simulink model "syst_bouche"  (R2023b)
settings: Solver=FixedStepAuto  StartTime=0.0  StopTime=15  FixedStep=0.0001  RelTol=1e-3
libraries: fl_lib x15, nesl_utility x9, ee_lib x1, sdl_lib x1

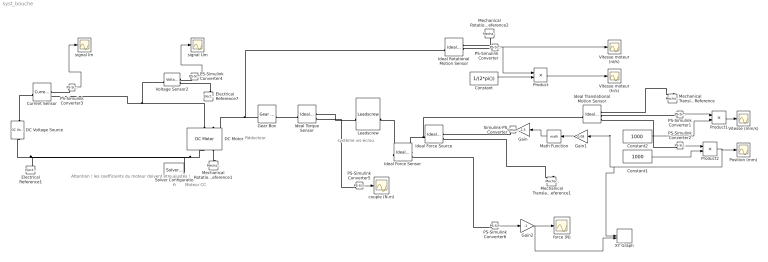
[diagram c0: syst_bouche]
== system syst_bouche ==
  note: Attention ! les coefficients du moteur doivent être ajustés !
  note: système vis-écrou
  note: Moteur CC
  note: Réducteur
  Constant : Constant  Value=1/(2*pi())
  Constant1 : Constant  Value=1000
  Constant2 : Constant  Value=1000
  Current Sensor : fl_lib/Electrical/Electrical Sensors/Current Sensor
  DC Motor : ee_lib/Electromechanical/Brushed Motors/DC Motor  field_option=ee.enum.field_option.pm  Rf=100 Ohm  Lf=1 H  Laf=0.15 H  If0=0 A  parameterization=ee.enum.dcparam_option.circuit_param  Ra=2.22 Ohm  La=0.1e-3 H  emf_or_torque=ee.enum.emf_or_torque.kv  Kv=0.0113 V/(rad/s)  Ki=0.01 N*m/A  T_stall=0.24e-3 N*m  w_max=19100 rpm  w_rated=15000 rpm  P_rated=0.08 W  V_rated=1.5 V  lam_param=ee.enum.lam_param.damping  i_noload=0 A  V_i_noload=1.5 V  J=50 g*cm^2  lam=0.0000015 N*m/(rad/s)  speed0=0 rpm  enable_fault_armature=simscape.enum.onoff.off  rev_faulted=1 / 3  G_faulted_armature=1e-5 S  fault_trigger_armature=ee.enum.faults.faultTrigger.temporal  t_fault_armature=1 s  max_permissible_current_armature=inf A  t_fail_on_current_armature=1 s  enable_fault_field=simscape.enum.onoff.off  G_faulted_field=1e-5 S  fault_trigger_field=ee.enum.faults.faultTrigger.temporal  t_fault_field=1 s  max_permissible_current_field=inf A  t_fail_on_current_field=1 s  fault_action=simscape.enum.assert.action.none  alpha=3.93e-3 1/K  Tmeas=25 degC  thermal_mass=100 J/K  initial_temperature=25 degC
  DC Voltage Source : fl_lib/Electrical/Electrical Sources/DC Voltage Source  v0=12 V
  Electrical Reference1 : fl_lib/Electrical/Electrical Elements/Electrical Reference
  Electrical Reference7 : fl_lib/Electrical/Electrical Elements/Electrical Reference
  Gain : Gain  Gain=2.3
  Gain1 : Gain  Gain=0.08
  Gain2 : Gain  Gain=-1
  Gear Box : fl_lib/Mechanical/Mechanisms/Gear Box  ratio=1  t_in_specify=off  t_in_priority=None  t_in=0 N*m  t_in_nominal_specify=off  t_in_nominal_unit=N*m  t_in_nominal_value=1  t_out_specify=off  t_out_priority=None  t_out=0 N*m  t_out_nominal_specify=off  t_out_nominal_unit=N*m  t_out_nominal_value=1
  Ideal Force Sensor : fl_lib/Mechanical/Mechanical Sensors/Ideal Force Sensor
  Ideal Force Source : fl_lib/Mechanical/Mechanical Sources/Ideal Force Source
  Ideal Rotational Motion Sensor : fl_lib/Mechanical/Mechanical Sensors/Ideal Rotational Motion Sensor  reference=foundation.enum.MeasurementReference.difference  acceleration_port=false  velocity_port=true  position_port=true  wrap_angle=simscape.enum.onoff.off  offset=0 rad
  Ideal Torque Sensor : fl_lib/Mechanical/Mechanical Sensors/Ideal Torque Sensor
  Ideal Translational Motion Sensor : fl_lib/Mechanical/Mechanical Sensors/Ideal Translational Motion Sensor  reference=foundation.enum.MeasurementReference.difference  acceleration_port=false  velocity_port=true  position_port=true  offset=0 m
  Leadscrew : sdl_lib/Gears/Rotational- Translational/Leadscrew  Lead=0 mm  helix_type=sdl.enum.handedness.right  friction_model=sdl.enum.gear_friction.constant  friction_parameterization=sdl.enum.frictionParameterization.geometry  lambda=15 deg  alpha=14.5 deg  fr_coeff=0.08  eff_sn=0.75  eff_ns=0.45  temperature_TLU=[280, 300, 320] K  efficiency_sn_TLU=[.75, .65, .6]  efficiency_ns_TLU=[.5, .45, .4]  pwr_thr=0.001 W  mu_visc=0 N*m/(rad/s)  thermal_mass=50 J/K  temperature_specify=off  temperature_priority=High  temperature=300 K  temperature_nominal_specify=off  temperature_nominal_unit=K  temperature_nominal_value=1
  Math Function : Math
  Mechanical Rotational Reference1 : fl_lib/Mechanical/Rotational Elements/Mechanical Rotational Reference
  Mechanical Rotational Reference2 : fl_lib/Mechanical/Rotational Elements/Mechanical Rotational Reference
  Mechanical Translational Reference : fl_lib/Mechanical/Translational Elements/Mechanical Translational Reference
  Mechanical Translational Reference1 : fl_lib/Mechanical/Translational Elements/Mechanical Translational Reference
  PS-Simulink Converter{,1..6} (7 alike) : nesl_utility/PS-Simulink Converter  PhysicalDomain=network_engine_domain  SubClassName=ps_output  LeftPortType=input  RightPortType=output  PseudoPeriodic=off  Frequencies=[]  VectorFormat=1-D array  Unit=inherit  AffineConversion=off
  Position (mm) : Scope
  Product : Product
  Product1 : Product
  Product2 : Product
  Simulink-PS Converter : nesl_utility/Simulink-PS Converter  PhysicalDomain=network_engine_domain  SubClassName=ps_input  LeftPortType=input  RightPortType=output  PseudoPeriodic=off  Frequencies=[]  NoiseDistribution=none  NoiseParameters=[]  Unit=1  AffineConversion=off  FilteringAndDerivatives=provide  SimscapeFilterOrder=1  InputFilterTimeConstant=0.001  UdotUserProvided=0
  Solver Configuration : nesl_utility/Solver Configuration  PhysicalDomain=network_engine_domain  SubClassName=solver  LeftPortType=input  RightPortType=generic  Tones=[]  Harmonics=[]  SimulateNoise=off  Profile=off  UseLocalSampling=off  EnableSwitchedLinearOptims=on  FrequencyDomain=off  UseCCode=off  RelTol=0.001  AbsTol=1e-06  MinStep=1e-09  ToWorkspace=off  RevertToSquareIcSolve=off  NumHomotopyIterations=100  PhasorMode=off  PhasorModeNumHarmonics=1  ConsistencySolver=NEWTON_FTOL  IndexReductionMethod=DerivativeReplacement  DoDC=off  ResidualTolerance=1e-09  ConsistencyTolSource=GLOBAL  ConsistencyAbsTol=0.001  ConsistencyRelTol=0.001  ConsistencyTolFactor=0.001  UseLocalSolver=off  LocalSolverChoice=NE_BACKWARD_EULER_ADVANCER  ResolveIndetEquations=on  FunctionEvalNumThread=1  LocalSolverSampleTime=0.001  DoFixedCost=off  MaxNonlinIter=3  MaxModeIter=2  ComputeImpulses=off  ImpulseIterations=2  LinearAlgebra=Full  LinearAlgebraNumThread=0  EquationFormulation=NE_TIME_EF  DelaysMemoryBudget=1024  AutomaticFiltering=on  FilteringTimeConstant=0.001  PartitionStorageMethod=AS_NEEDED  PartitionMemoryBudget=1024  PartitionMethod=FAST  MultibodyUseLocalSolver=off  MultibodyLocalSolverChoice=ODE1  MultibodyLocalSolverSampleTime=0.001
  Vitesse (mm/s) : Scope
  Vitesse moteur (rd/s) : Scope
  Vitesse moteur (tr/s) : Scope
  Voltage Sensor2 : fl_lib/Electrical/Electrical Sensors/Voltage Sensor
  XY Graph : Record  FileSettingsInternal="{\"entries\":[{\"content\":{\"excelSettings\":{\"content\":{},\"type\":\"Streamout.ExcelSettings\"}},\"type\":\"Streamout.FileSettingStorage\",\"uuid\":\"\"}],\"packageUris\":[\"http:\\/\\/schema.mathworks.com\\/mf0\\/streamout_blocks\\/R2020a\"],\"version\":\"1.0\"}"  Layout=[1 1]  SignalsInternal="{\"entries\":[{\"content\":{\"signals\":[{\"content\":{\"blockPath\":[],\"dimensions\":[1],\"domain\":\"\",\"lineColor\":\"#a2142f\",\"plots\":[1],\"port\":1,\"signalID\":300732,\"signalName\":\"Product2\"},\"type\":\"RecordBlkView.Signal\",\"uuid\":\"\"},{\"content\":{\"blockPath\":[],\"dimensions\":[1],\"domain\":\"\",\"lineColor\":\"#139fff\",\"plots\":[1],\"port\":2,\"signalID\":300735,\"signalName\":\"Gain2\"},\"type\":\"RecordBlkView.Signal\",\"uuid\":\"\"}]},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"  VisualizationBindings="{\"xyplotplugin\":{\"info\":[{\"series\":[{\"bindingParametersList\":[{\"parameter\":\"X-Axis\",\"signalID\":300732,\"signalName\":\"Product2\"},{\"parameter\":\"Y-Axis\",\"signalID\":300735,\"signalName\":\"Gain2\"}],\"seriesID\":19179}],\"subplotID\":1}]}}"  CompatibilityTag=XY
  couple (N.m) : Scope
  force (N) : Scope
  signal Im : Scope
  signal Um : Scope
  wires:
  Product1/1 -> Vitesse (mm/s)/1
  Product/1 -> Vitesse moteur (tr/s)/1
  Constant/1 -> Product/2
  PS-Simulink Converter/1 -> Vitesse moteur (rd/s)/1, Product/1
  Constant2/1 -> Product1/2
  Constant1/1 -> Product2/2
  PS-Simulink Converter1/1 -> Product1/1
  PS-Simulink Converter4/1 -> signal Um/1
  PS-Simulink Converter2/1 -> Product2/1
  PS-Simulink Converter3/1 -> signal Im/1
  PS-Simulink Converter5/1 -> couple (N.m)/1
  Gain/1 -> Simulink-PS Converter/1
  Math Function/1 -> Gain/1
  Gain1/1 -> Math Function/1
  Product2/1 -> Position (mm)/1, XY Graph/1, Gain1/1
  PS-Simulink Converter6/1 -> Gain2/1
  Gain2/1 -> XY Graph/2, force (N)/1
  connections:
  DC Motor/RConn1 -- Solver Configuration/RConn1 -- Electrical Reference1/LConn1 -- DC Voltage Source/RConn1
  DC Motor/LConn1 -- Current Sensor/RConn2 -- Voltage Sensor2/LConn1
  Electrical Reference7/LConn1 -- Voltage Sensor2/RConn2
  DC Motor/RConn2 -- Mechanical Rotational Reference1/LConn1
  Ideal Translational Motion Sensor/RConn1 -- Mechanical Translational Reference/LConn1
  Ideal Translational Motion Sensor/RConn3 -- PS-Simulink Converter2/LConn1
  Ideal Translational Motion Sensor/RConn2 -- PS-Simulink Converter1/LConn1
  PS-Simulink Converter4/LConn1 -- Voltage Sensor2/RConn1
  Ideal Rotational Motion Sensor/RConn2 -- PS-Simulink Converter/LConn1
  Mechanical Rotational Reference2/LConn1 -- Ideal Rotational Motion Sensor/RConn1
  Ideal Rotational Motion Sensor/LConn1 -- Gear Box/LConn1 -- DC Motor/LConn2
  PS-Simulink Converter3/LConn1 -- Current Sensor/RConn1
  DC Voltage Source/LConn1 -- Current Sensor/LConn1
  PS-Simulink Converter5/LConn1 -- Ideal Torque Sensor/RConn2
  Gear Box/RConn1 -- Ideal Torque Sensor/LConn1
  Ideal Torque Sensor/RConn1 -- Leadscrew/LConn1
  Ideal Translational Motion Sensor/LConn1 -- Ideal Force Sensor/RConn1 -- Ideal Force Source/LConn1
  Ideal Force Source/RConn2 -- Mechanical Translational Reference1/LConn1
  PS-Simulink Converter6/LConn1 -- Ideal Force Sensor/RConn2
  Simulink-PS Converter/RConn1 -- Ideal Force Source/RConn1
  Ideal Force Sensor/LConn1 -- Leadscrew/RConn1
